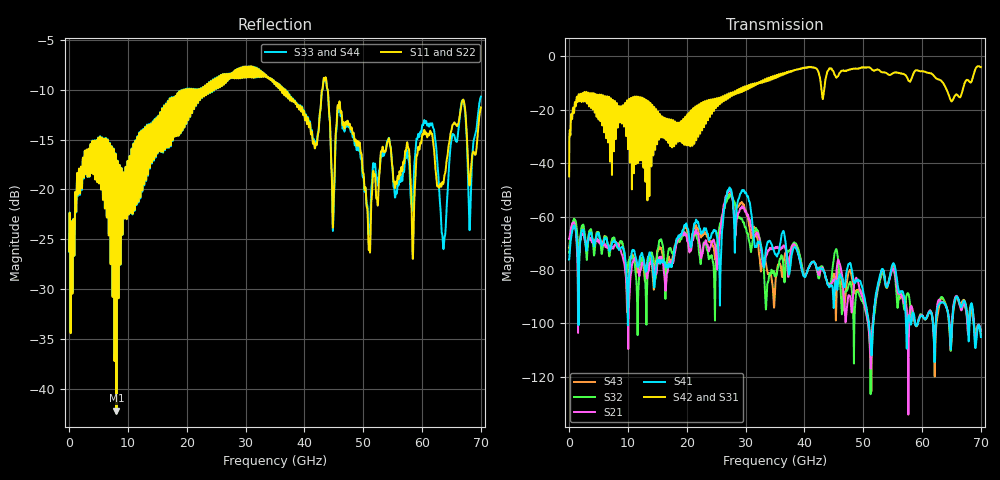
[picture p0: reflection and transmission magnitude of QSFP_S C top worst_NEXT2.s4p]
! AWR Design Environment (8415) Tue Jan 08 12:57:41 2019
! Document = 'QSFP Channel_S'
! nPorts: 4, nXvals: 7001
# HZ S DB R 50
!Freq DBS11 AngS11 DBS12 AngS12 DBS13 AngS13 DBS14 AngS14
!	DBS21 AngS21 DBS22 AngS22 DBS23 AngS23 DBS24 AngS24
!	DBS31 AngS31 DBS32 AngS32 DBS33 AngS33 DBS34 AngS34
!	DBS41 AngS41 DBS42 AngS42 DBS43 AngS43 DBS44 AngS44
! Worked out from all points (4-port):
!   7000 points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, 10 MHz to 70 GHz, reference 50 ohm
!   strongest paths, dB at 10 MHz, 17.51 GHz, 35.01 GHz, 52.51 GHz, 70 GHz:
!     S42: -45.0, -33.1, -7.3, -5.0, -4.0
!     S31: -44.8, -33.9, -7.3, -5.0, -4.0
!     S41: -76.1, -77.9, -74.1, -85.0, -105.1
!     S21: -68.4, -77.5, -71.9, -85.8, -102.9
!     S32: -73.5, -73.4, -82.1, -87.0, -102.3
!     S43: -71.7, -76.4, -88.0, -86.1, -104.5
!   lowest |S11| = -42.2 dB at 8.06 GHz (marker M1), VSWR 1.02, Z = 49.9 - j0.765 ohm
!   |S11| at or under -10 dB: start of sweep to 19.42 GHz; 36.78 GHz to 43.01 GHz (6.234 GHz wide, 15.6 % of centre); 43.97 GHz to end of sweep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
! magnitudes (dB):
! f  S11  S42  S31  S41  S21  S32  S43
! 10 MHz  -26.2  -45.0  -44.8  -76.1  -68.4  -73.5  -71.7
! 1.63 GHz  -18.8  -14.2  -14.4  -91.8  -78.1  -75.0  -80.3
! 8.06 GHz  -42.2  -18.4  -18.4  -70.2  -69.8  -70.6  -69.9
! 24.66 GHz  -10.0  -18.7  -18.7  -65.1  -69.2  -83.6  -72.6
! 27.27 GHz  -8.8  -15.1  -15.1  -49.1  -49.8  -51.9  -51.4
! 33.98 GHz  -8.9  -8.0  -8.0  -69.3  -72.7  -82.4  -81.2
! 70 GHz  -11.8  -4.0  -4.0  -105.1  -102.9  -102.3  -104.5
